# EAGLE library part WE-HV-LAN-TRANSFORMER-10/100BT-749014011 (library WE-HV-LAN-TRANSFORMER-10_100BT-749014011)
WE-LAN HV LAN-Transformer Characteristics: •Compliant with IEEE802.3 and 802.3af standards •Operating temperature: 0 °C to +70 °C •SMD •4 kV Hipot test Applications: •Ethernet •Compliant with most IC's for Ethernet applications like Intel, AMD, Conexant, Realtek, etc. •Hub, Router, Switches, medical applications
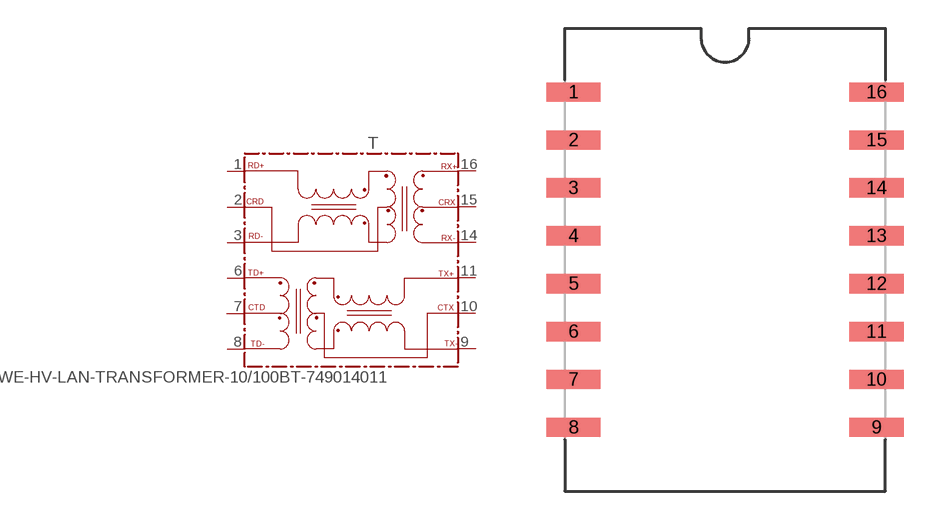
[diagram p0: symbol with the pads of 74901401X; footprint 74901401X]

Designator prefix T

## WE-HV-LAN-TRANSFORMER-10/100BT-749014011 (MPN: 749014011; OC_FARNELL: 1961662; OC_NEWARK: 61T8050; PACKAGE: 10/100/BT with CMC; SUPPLIER: Wuerth Elektronik)  [74901401X]
1  RD+
2  CRD
3  RD-
6  TD+
7  CTD
8  TD-
9  TX-
10  CTX
11  TX+
14  RX-
15  CRX
16  RX+

## Footprint 74901401X (pad centres in mm)
MAX Height=10.85 mm
smd 2.87 x 1.02: 1 -8.03,8.89; 2 -8.03,6.35; 3 -8.03,3.81; 4 -8.03,1.27; 5 -8.03,-1.27; 6 -8.03,-3.81; 7 -8.03,-6.35; 8 -8.03,-8.89; 9 8.03,-8.89; 10 8.03,-6.35; 11 8.03,-3.81; 12 8.03,-1.27; 13 8.03,1.27; 14 8.03,3.81; 15 8.03,6.35; 16 8.03,8.89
